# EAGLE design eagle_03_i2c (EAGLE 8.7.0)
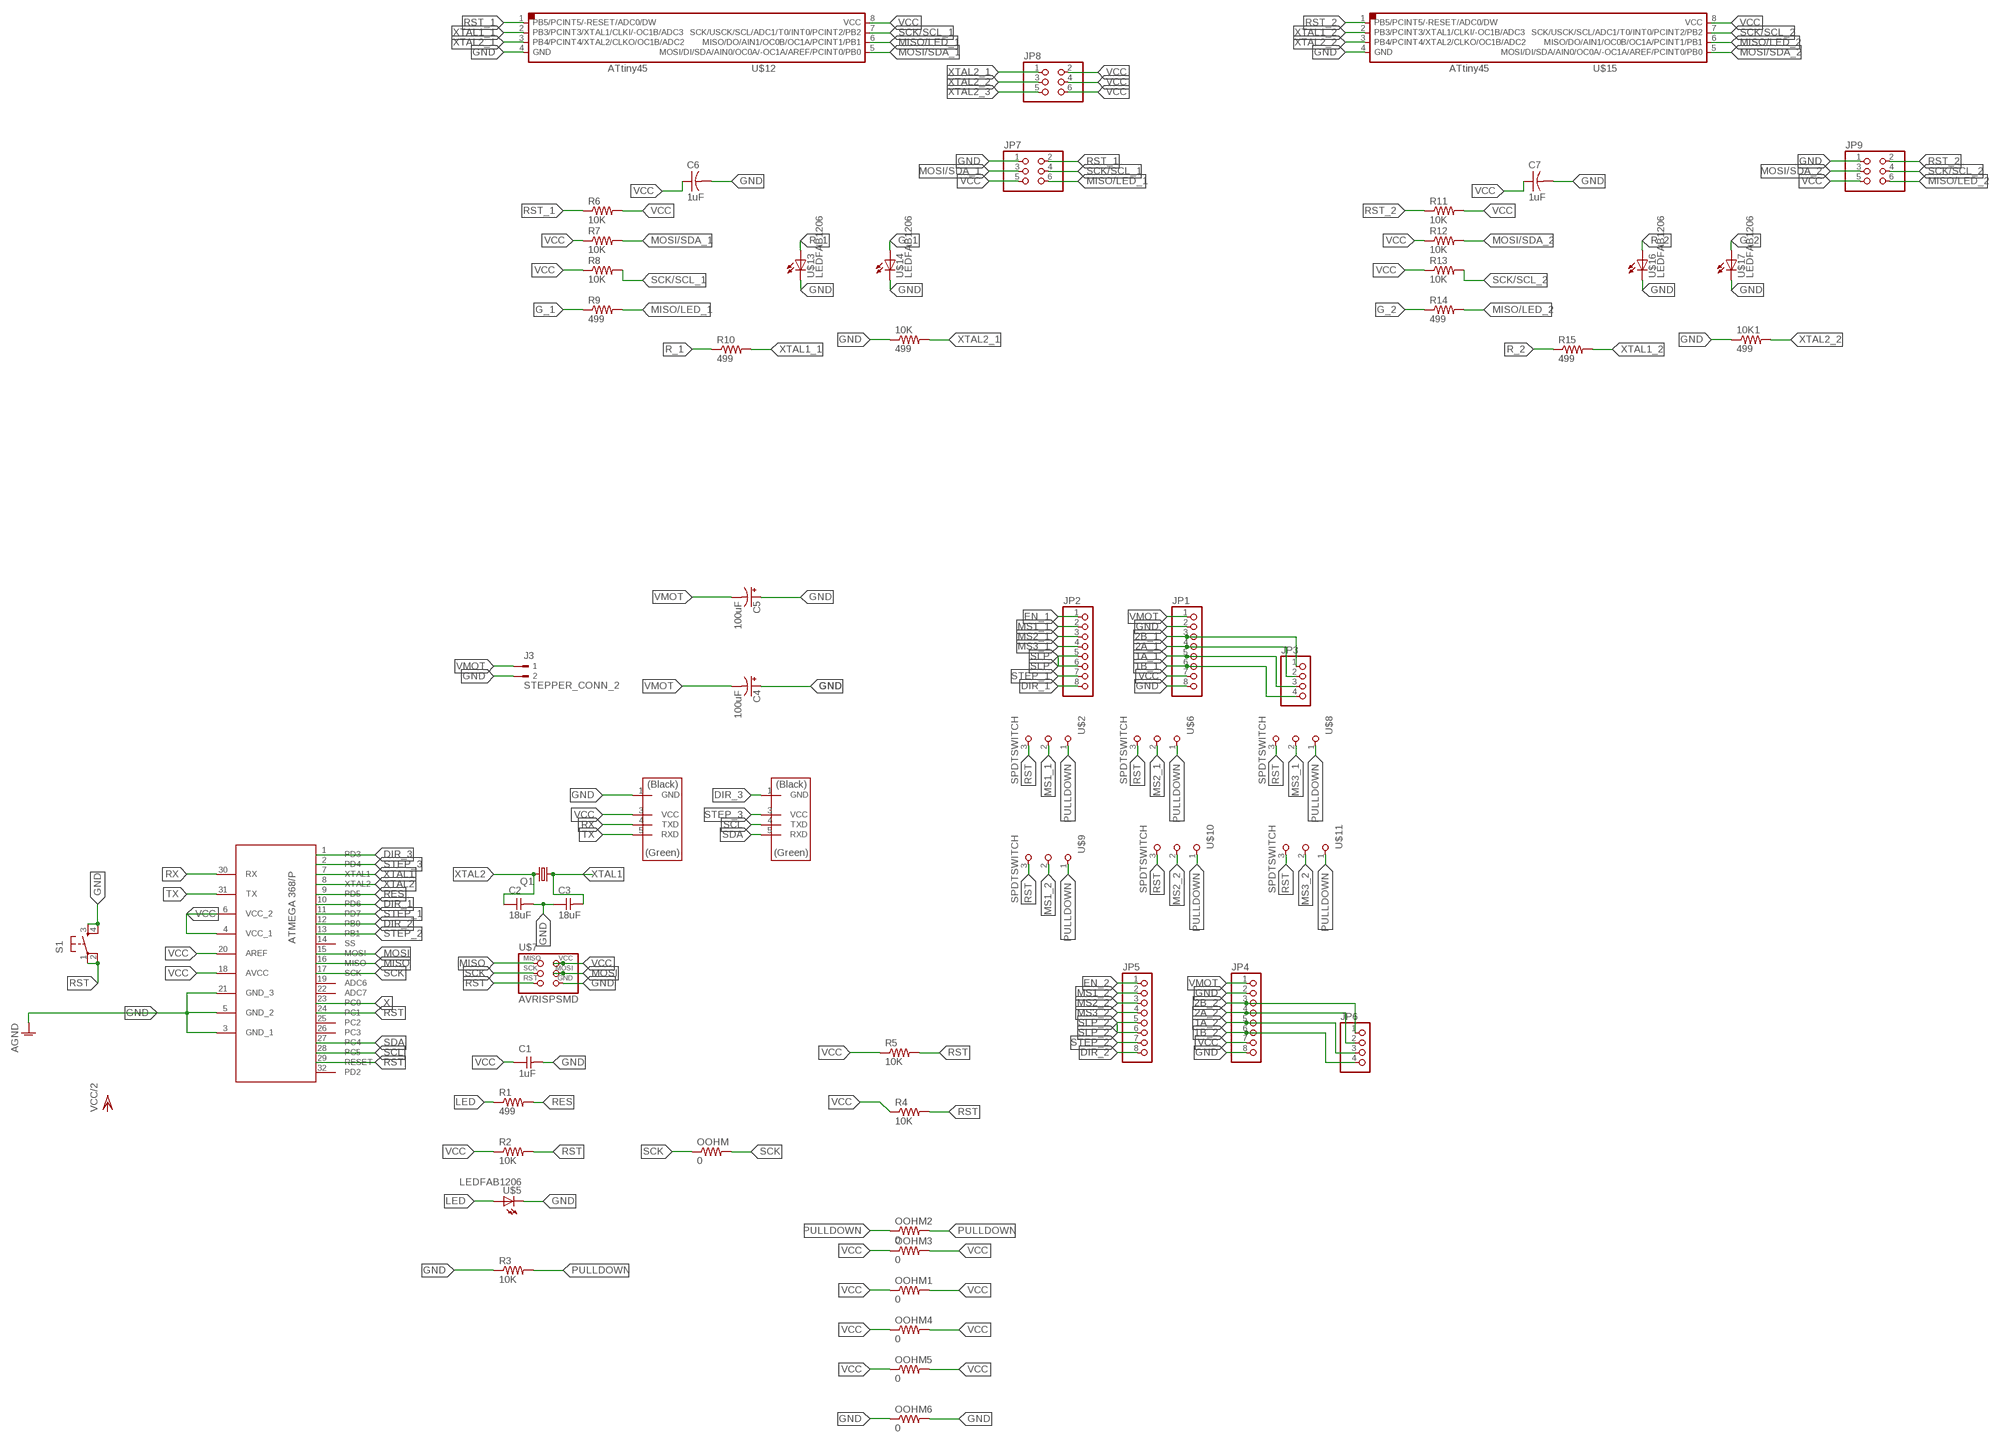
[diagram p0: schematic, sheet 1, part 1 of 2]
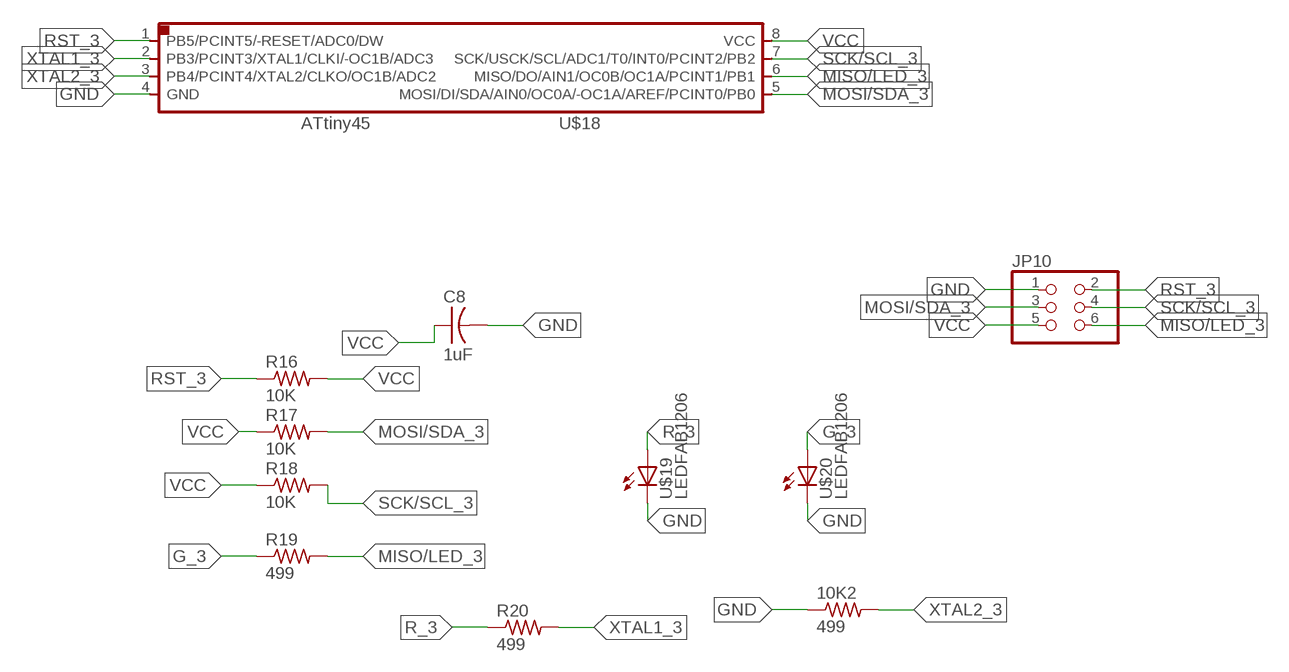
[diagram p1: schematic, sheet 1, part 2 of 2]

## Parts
10K  499  RES-US1206FAB  [R1206FAB]
10K1  499  RES-US1206FAB  [R1206FAB]
10K2  499  RES-US1206FAB  [R1206FAB]
C1  1uF  CAP-UNPOLARIZEDFAB  [C1206FAB]
C2  18uF  CAP-UNPOLARIZEDFAB  [C1206FAB]
C3  18uF  CAP-UNPOLARIZEDFAB  [C1206FAB]
C4  100uF  CAP_POLC  [PANASONIC_C]
C5  100uF  CAP_POLC  [PANASONIC_C]
C6  1uF  CAP-US1206FAB  [C1206FAB]
C7  1uF  CAP-US1206FAB  [C1206FAB]
C8  1uF  CAP-US1206FAB  [C1206FAB]
J3  STEPPER_CONN_2  PM5.08/2/90BLK  [WEIDMULLER_PM5.08_2]
JP1  PINHD-1X8  [1X08]
JP2  PINHD-1X8  [1X08]
JP3  PINHD-1X4  [1X04]
JP4  PINHD-1X8  [1X08]
JP5  PINHD-1X8  [1X08]
JP6  PINHD-1X4  [1X04]
JP7  PINHD-2X3-SMD  [2X03SMD]
JP8  PINHD-2X3-SMD  [2X03SMD]
JP9  PINHD-2X3-SMD  [2X03SMD]
JP10  PINHD-2X3-SMD  [2X03SMD]
OOHM  0  RES-US1206FAB  [R1206FAB]
OOHM1  0  RES-US1206FAB  [R1206FAB]
OOHM2  0  RES-US1206FAB  [R1206FAB]
OOHM3  0  RES-US1206FAB  [R1206FAB]
OOHM4  0  RES-US1206FAB  [R1206FAB]
OOHM5  0  RES-US1206FAB  [R1206FAB]
OOHM6  0  RES-US1206FAB  [R1206FAB]
Q1  CRYSTALSM49  [SM49]
R1  499  RES-US1206FAB  [R1206FAB]
R2  10K  RES-US1206FAB  [R1206FAB]
R3  10K  RES-US1206FAB  [R1206FAB]
R4  10K  RES-US1206FAB  [R1206FAB]
R5  10K  RES-US1206FAB  [R1206FAB]
R6  10K  RES-US1206FAB  [R1206FAB]
R7  10K  RES-US1206FAB  [R1206FAB]
R8  10K  RES-US1206FAB  [R1206FAB]
R9  499  RES-US1206FAB  [R1206FAB]
R10  499  RES-US1206FAB  [R1206FAB]
R11  10K  RES-US1206FAB  [R1206FAB]
R12  10K  RES-US1206FAB  [R1206FAB]
R13  10K  RES-US1206FAB  [R1206FAB]
R14  499  RES-US1206FAB  [R1206FAB]
R15  499  RES-US1206FAB  [R1206FAB]
R16  10K  RES-US1206FAB  [R1206FAB]
R17  10K  RES-US1206FAB  [R1206FAB]
R18  10K  RES-US1206FAB  [R1206FAB]
R19  499  RES-US1206FAB  [R1206FAB]
R20  499  RES-US1206FAB  [R1206FAB]
S1  6MM_SWITCH6MM_SWITCH  [6MM_SWITCH]
U$1  ATMEGA368  [ATMEGA328/P]
U$2  SPDTSWITCH  [SPDTSWITCH]
U$3  FTDI_2  [1X06SMD_2]
U$4  FTDI_2  [1X06SMD_2]
U$5  LEDFAB1206  [LED1206FAB]
U$6  SPDTSWITCH  [SPDTSWITCH]
U$7  AVRISPSMD  [2X03SMD]
U$8  SPDTSWITCH  [SPDTSWITCH]
U$9  SPDTSWITCH  [SPDTSWITCH]
U$10  SPDTSWITCH  [SPDTSWITCH]
U$11  SPDTSWITCH  [SPDTSWITCH]
U$12  ATTINY45SI  [SOIC8]
U$13  LEDFAB1206  [LED1206FAB]
U$14  LEDFAB1206  [LED1206FAB]
U$15  ATTINY45SI  [SOIC8]
U$16  LEDFAB1206  [LED1206FAB]
U$17  LEDFAB1206  [LED1206FAB]
U$18  ATTINY45SI  [SOIC8]
U$19  LEDFAB1206  [LED1206FAB]
U$20  LEDFAB1206  [LED1206FAB]

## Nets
1A_1: JP1.5 JP3.3
1A_2: JP4.5 JP6.3
1B_1: JP1.6 JP3.4
1B_2: JP4.6 JP6.4
2A_1: JP1.4 JP3.2
2A_2: JP4.4 JP6.2
2B_1: JP1.3 JP3.1
2B_2: JP4.3 JP6.1
DIR_1: JP2.8 U$1.10(PD6)
DIR_2: JP5.8 U$1.12(PB0)
DIR_3: U$1.1(PD3) U$3.1(GND)
EN_1: JP2.1
EN_2: JP5.1
G_1: R9.1 U$14.1(A)
G_2: R14.1 U$17.1(A)
G_3: R19.1 U$20.1(A)
GND: 10K1.1 10K2.1 10K.1 C1.2 C2.2 C3.1 C4.+ C5.+ C6.2 C7.2 C8.2 J3.2 JP1.2 JP1.8 JP4.2 JP4.8 JP7.1 JP9.1 JP10.1 OOHM6.1 OOHM6.2 R3.1 S1.3(S) S1.4(S1) U$1.3(GND_1) U$1.5(GND_2) U$1.21(GND_3) U$4.1(GND) U$5.2(C) U$7.6(GND) U$12.4(GND) U$13.2(C) U$14.2(C) U$15.4(GND) U$16.2(C) U$17.2(C) U$18.4(GND) U$19.2(C) U$20.2(C) ; supply symbol labelled AGND
LED: R1.1 U$5.1(A)
MISO: U$1.16(MISO) U$7.1(MISO)
MISO/LED_1: JP7.6 R9.2 U$12.6(MISO/DO/AIN1/OC0B/OC1A/PCINT1/PB1)
MISO/LED_2: JP9.6 R14.2 U$15.6(MISO/DO/AIN1/OC0B/OC1A/PCINT1/PB1)
MISO/LED_3: JP10.6 R19.2 U$18.6(MISO/DO/AIN1/OC0B/OC1A/PCINT1/PB1)
MOSI: U$1.15(MOSI) U$7.4(MOSI)
MOSI/SDA_1: JP7.3 R7.2 U$12.5(MOSI/DI/SDA/AIN0/OC0A/-OC1A/AREF/PCINT0/PB0)
MOSI/SDA_2: JP9.3 R12.2 U$15.5(MOSI/DI/SDA/AIN0/OC0A/-OC1A/AREF/PCINT0/PB0)
MOSI/SDA_3: JP10.3 R17.2 U$18.5(MOSI/DI/SDA/AIN0/OC0A/-OC1A/AREF/PCINT0/PB0)
MS1_1: JP2.2 U$2.2
MS1_2: JP5.2 U$9.2
MS2_1: JP2.3 U$6.2
MS2_2: JP5.3 U$10.2
MS3_1: JP2.4 U$8.2
MS3_2: JP5.4 U$11.2
PULLDOWN: OOHM2.1 OOHM2.2 R3.2 U$2.1 U$6.1 U$8.1 U$9.1 U$10.1 U$11.1
R_1: R10.1 U$13.1(A)
R_2: R15.1 U$16.1(A)
R_3: R20.1 U$19.1(A)
RES: R1.2 U$1.9(PD5)
RST: R2.2 R4.2 R5.2 S1.1(P) S1.2(P1) U$1.24(PC1) U$1.29(RESET) U$2.3 U$6.3 U$7.5(RST) U$8.3 U$9.3 U$10.3 U$11.3
RST_1: JP7.2 R6.1 U$12.1(PB5/PCINT5/-RESET/ADC0/DW)
RST_2: JP9.2 R11.1 U$15.1(PB5/PCINT5/-RESET/ADC0/DW)
RST_3: JP10.2 R16.1 U$18.1(PB5/PCINT5/-RESET/ADC0/DW)
RX: U$1.30(RX) U$4.4(TXD)
SCK: OOHM.1 OOHM.2 U$1.17(SCK) U$7.3(SCK)
SCK/SCL_1: JP7.4 R8.2 U$12.7(SCK/USCK/SCL/ADC1/T0/INT0/PCINT2/PB2)
SCK/SCL_2: JP9.4 R13.2 U$15.7(SCK/USCK/SCL/ADC1/T0/INT0/PCINT2/PB2)
SCK/SCL_3: JP10.4 R18.2 U$18.7(SCK/USCK/SCL/ADC1/T0/INT0/PCINT2/PB2)
SCL: U$1.28(PC5) U$3.4(TXD)
SDA: U$1.27(PC4) U$3.5(RXD)
SLP: JP2.5 JP2.6
SLP_2: JP5.5 JP5.6
STEP_1: JP2.7 U$1.11(PD7)
STEP_2: JP5.7 U$1.13(PB1)
STEP_3: U$1.2(PD4) U$3.3(VCC)
TX: U$1.31(TX) U$4.5(RXD)
VCC: C1.1 C6.1 C7.1 C8.1 JP1.7 JP4.7 JP7.5 JP8.2 JP8.4 JP8.6 JP9.5 JP10.5 OOHM1.1 OOHM1.2 OOHM3.1 OOHM3.2 OOHM4.1 OOHM4.2 OOHM5.1 OOHM5.2 R2.1 R4.1 R5.1 R6.2 R7.1 R8.1 R11.2 R12.1 R13.1 R16.2 R17.1 R18.1 U$1.4(VCC_1) U$1.6(VCC_2) U$1.18(AVCC) U$1.20(AREF) U$4.3(VCC) U$7.2(VCC) U$12.8(VCC) U$15.8(VCC) U$18.8(VCC)
VMOT: C4.- C5.- J3.1 JP1.1 JP4.1
X: U$1.23(PC0)
XTAL1: C3.2 Q1.1 U$1.7(XTAL1)
XTAL1_1: R10.2 U$12.2(PB3/PCINT3/XTAL1/CLKI/-OC1B/ADC3)
XTAL1_2: R15.2 U$15.2(PB3/PCINT3/XTAL1/CLKI/-OC1B/ADC3)
XTAL1_3: R20.2 U$18.2(PB3/PCINT3/XTAL1/CLKI/-OC1B/ADC3)
XTAL2: C2.1 Q1.2 U$1.8(XTAL2)
XTAL2_1: 10K.2 JP8.1 U$12.3(PB4/PCINT4/XTAL2/CLKO/OC1B/ADC2)
XTAL2_2: 10K1.2 JP8.3 U$15.3(PB4/PCINT4/XTAL2/CLKO/OC1B/ADC2)
XTAL2_3: 10K2.2 JP8.5 U$18.3(PB4/PCINT4/XTAL2/CLKO/OC1B/ADC2)
Unconnected: U$1.14(SS) U$1.19(ADC6) U$1.22(ADC7) U$1.25(PC2) U$1.26(PC3) U$1.32(PD2)

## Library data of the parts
10K 10K1 10K2 R6-R20 = 01fab:RES-US: Resistor (US Symbol)
C1-C3 = fab:CAP-UNPOLARIZED
C4 C5 = SparkFun-Capacitors:CAP_POL: Capacitor Polarized
C6-C8 = 01fab:CAP-US
J3 = WEIDMULLER-PM5.08_2_90BLK:PM5.08/2/90BLK: TERMINAL BLOCK, SIDE ENTRY, 2WAY; MPN: PM5.08/2/90 BLK; OC_FARNELL: 1131855; OC_NEWARK: 26M1980; PACKAGE: TH-R/A; SUPPLIER: WEIDMULLER
JP1 JP2 JP4 JP5 = pinhead:PINHD-1X8: PIN HEADER
JP3 JP6 = pinhead:PINHD-1X4: PIN HEADER
JP7-JP10 = 01fab:PINHD-2X3-SMD: PIN HEADER
OOHM OOHM1-OOHM6 R1-R5 = fab:RES-US: Resistor (US Symbol)
Q1 = crystal:CRYSTAL: CRYSTAL; OC_FARNELL: unknown; OC_NEWARK: unknown
S1 = fab:6MM_SWITCH: OMRON SWITCH
U$1 = Paul:ATMEGA368
U$2 U$6 U$8-U$11 = 01fab:SPDTSWITCH
U$3 = 01fab:FTDI_2
U$4 = fab:FTDI_2
U$5 = fab:LED: LED
U$7 = 01fab:AVRISP
U$12 U$15 U$18 = 01fab:ATTINY45
U$13 U$14 U$16 U$17 U$19 U$20 = 01fab:LED: LED

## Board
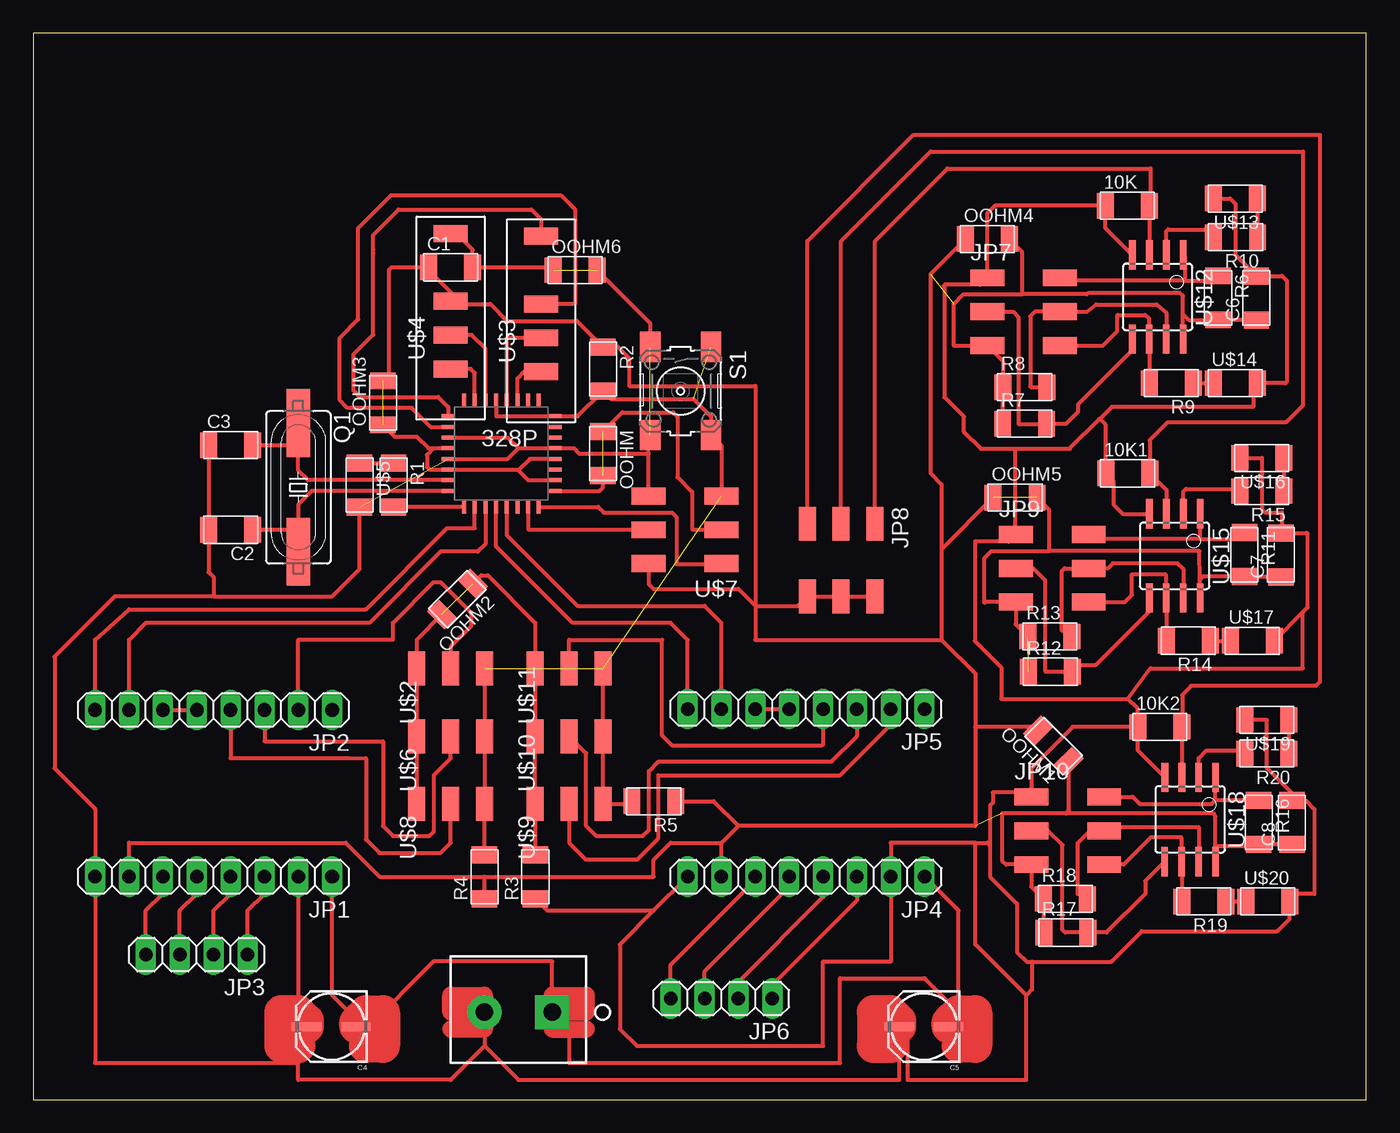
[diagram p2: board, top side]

Size 100 x 80 mm. Coordinates in mm from the lower left corner, seen from the top.
Outline: 0,0 100,0 100,80 0,80 0,0
Copper layers (1*16): Top 0.035mm / dielectric 1.5mm / Bottom 0.035mm
Design rules "default *": minimum track width 6mil, minimum drill 0.35mm, track to track 16mil, track to pad 16mil, pad to pad 16mil, via to via 16mil, smd to smd 16mil, copper to edge 40mil, drill to drill 6mil, minimum pad ring 10mil, minimum via ring 8mil, stop-mask expansion 4mil, vias tented up to drill 0mil, thermal gap 10mil

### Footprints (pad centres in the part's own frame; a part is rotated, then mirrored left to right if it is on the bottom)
R1206FAB = smd 1.27 x 1.905: 1 -1.651,0; 2 1.651,0
C1206FAB = smd 1.27 x 1.905: 1 -1.651,0; 2 1.651,0
PANASONIC_C = smd 2.2 x 0.65: + 1.9,-0.2; - -1.8,-0.2
WEIDMULLER_PM5.08_2 = drill 1.3 pad 2.54 square: 1 -2.54,0 | drill 1.3 pad 2.54: 2 2.54,0
1X08 = drill 1.016 long: 1 -8.89,0; 2 -6.35,0; 3 -3.81,0; 4 -1.27,0; 5 1.27,0; 6 3.81,0; 7 6.35,0; 8 8.89,0
1X04 = drill 1.016 long: 1 -3.81,0; 2 -1.27,0; 3 1.27,0; 4 3.81,0
2X03SMD = smd 2.54 x 1.27: 1 -2.54,2.54; 2 2.92,2.54; 3 -2.54,0; 4 2.92,0; 5 -2.54,-2.54; 6 2.92,-2.54
SM49 = smd 5.08 x 1.778: 1 -4.826,0; 2 4.826,0
6MM_SWITCH = smd 2.286 x 1.524: 1 -3.302,2.286; 2 3.302,2.286; 3 -3.302,-2.286; 4 3.302,-2.286
ATMEGA328/P = smd 1 x 0.3: 1 -4,2.8; 2 -4,2; 3 -4,1.2; 4 -4,0.4; 5 -4,-0.4; 6 -4,-1.2; 7 -4,-2; 8 -4,-2.8; 17 4,-2.8; 18 4,-2; 19 4,-1.2; 20 4,-0.4; 21 4,0.4; 22 4,1.2; 23 4,2; 24 4,2.8 | smd 0.3 x 1: 9 -2.8,-4; 10 -2,-4; 11 -1.2,-4; 12 -0.4,-4; 13 0.4,-4; 14 1.2,-4; 15 2,-4; 16 2.8,-4; 25 2.8,4; 26 2,4; 27 1.2,4; 28 0.4,4; 29 -0.4,4; 30 -1.2,4; 31 -2,4; 32 -2.8,4
SPDTSWITCH = smd 2.54 x 1.27: 1 0.38,2.54; 2 0.38,0; 3 0.38,-2.54
1X06SMD_2 = smd 2.54 x 1.27: 1 0,6.35; 3 0,1.27; 4 0,-1.27; 5 0,-3.81
LED1206FAB = smd 1.27 x 1.905: 1 -1.651,0; 2 1.651,0
SOIC8 = smd 0.5 x 2.2: 1 -1.905,-3.154; 2 -0.645,-3.154; 3 0.625,-3.154; 4 1.895,-3.154; 5 1.905,3.154; 6 0.635,3.154; 7 -0.635,3.154; 8 -1.905,3.154

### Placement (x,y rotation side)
10K  82.09,67.06 0 top
10K1  82.1,46.98 0 top
10K2  84.52,27.96 0 top
C1  31.31,62.44 0 top
C2  14.8,42.75 180 top
C3  14.8,49.1 0 top
C4  22.42,5.29 180 top
C5  66.87,5.29 180 top
C6  91.75,60.15 90 top
C7  93.61,40.87 90 top
C8  94.43,20.78 90 top
J3  36.39,6.56 180 top
JP1  13.53,16.72 180 top
JP2  13.53,29.23 180 top
JP3  12.26,10.87 180 top
JP4  57.98,16.72 180 top
JP5  57.98,29.3 180 top
JP6  51.63,7.57 180 top
JP7  74.11,59.11 0 top
JP8  60.61,40.66 270 top
JP9  76.26,39.86 0 top
JP10  77.42,20.17 0 top
OOHM  42.74,48.47 270 top
OOHM1  76.54,26.52 135 top
OOHM2  31.82,37.54 225 top
OOHM3  26.23,52.28 90 top
OOHM4  71.58,64.56 0 top
OOHM5  73.66,45.16 0 top
OOHM6  40.64,62.23 0 top
Q1  19.88,45.93 270 top
R1  27.03,46.1 270 top
R2  42.74,54.82 270 top
R3  37.66,16.72 90 top
R4  33.85,16.72 90 top
R5  46.55,22.38 180 top
R6  88.89,60.15 270 top
R7  74.38,50.71 0 top
R8  74.38,53.45 0 top
R9  85.37,53.76 180 top
R10  90.2,64.7 180 top
R11  90.87,40.88 270 top
R12  76.32,32.1 0 top
R13  76.28,34.74 0 top
R14  86.65,34.43 180 top
R15  92.16,45.66 180 top
R16  91.94,20.8 270 top
R17  77.46,12.53 0 top
R18  77.44,15.05 0 top
R19  87.82,14.86 180 top
R20  92.55,25.95 180 top
S1  48.56,53.16 270 top
U$1  35.12,48.47 0 top
U$2  31.31,31.96 90 top
U$3  38.1,58.42 0 top
U$4  31.31,58.63 0 top
U$5  24.47,46.1 270 top
U$6  31.31,26.88 90 top
U$7  49.09,42.75 180 top
U$8  31.31,21.8 90 top
U$9  40.2,21.8 90 top
U$10  40.2,26.88 90 top
U$11  40.2,31.96 90 top
U$12  84.36,60.21 180 top
U$13  90.19,67.6 180 top
U$14  90.17,53.75 0 top
U$15  85.63,40.79 180 top
U$16  92.17,48.14 180 top
U$17  91.45,34.42 0 top
U$18  86.79,21.01 180 top
U$19  92.54,28.48 180 top
U$20  92.61,14.86 0 top

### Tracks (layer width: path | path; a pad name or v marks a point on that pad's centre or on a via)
1A_1
  Top 0.305: 10.99,11.59 10.99,14.18 12.26,15.45 JP1.5
  Top 1.27: 12.19,17.46 12.26,17.39 JP1.5 | JP3.3 10.99,11.59
1A_2
  Top 0.305: 50.36,8.03 50.36,9.6 56.71,15.95
  Top 1.27: JP6.3 50.36,8.03 | JP4.5 56.71,15.95
1B_1
  Top 0.305: 8.45,11.59 8.45,14.18 9.72,15.45 9.72,16.27
  Top 1.27: JP1.6 9.72,16.27 | JP3.4 8.45,11.59
1B_2
  Top 0.305: 47.82,8.38 47.82,10.11 54.07,16.37
  Top 1.27: 47.88,6.77 47.82,6.84 JP6.4 47.82,8.38 | JP4.6 54.07,16.62 54.07,16.37
2A_1
  Top 0.305: 13.53,11.73 13.53,14.18 14.8,15.45 JP1.4
  Top 1.27: JP1.4 14.77,16.74 14.77,17.39 | JP3.2 13.53,11.73
2A_2
  Top 0.305: 59.25,16.06 59.25,15.19 52.9,8.84 52.9,7.89
  Top 1.27: JP6.2 52.9,7.89 | JP4.4 59.25,16.06
2B_1
  Top 0.305: 16.07,11.38 16.07,14.18 17.34,15.45 JP1.3
  Top 1.27: JP1.3 17.34,17.58 17.36,17.6 | JP3.1 16.07,11.38
2B_2
  Top 0.305: 61.79,16.34 61.79,14.94 55.44,8.59 55.44,7.82
  Top 1.27: JP6.1 55.44,7.82 | JP4.3 61.79,16.34
DIR_1
  Top 0.305: U$1.10 33.12,42.88 31.05,42.88 24.96,36.78 7.18,36.78 4.64,34.5 4.64,29.54
  Top 1.27: JP2.8 4.64,29.54
DIR_2
  Top 0.305: 49.09,29.61 49.09,34.5 47.82,35.77 40.47,35.77 34.72,41.51 U$1.12
  Top 1.27: JP5.8 49.09,29.61
DIR_3
  Top 0.305: U$1.1 31.12,51.96 30.37,52.71 24.48,52.71 24,53.22 24,55.88 25.5,57.38 25.5,63.5 25.5,63.8 25.5,64.87 27.4,66.77 37.37,66.77 38.1,66.04 U$3.1
EN_1
  Top 1.27: JP2.1 22.42,28.74 22.46,28.7
EN_2
  Top 1.27: JP5.1 66.95,29.22 66.95,28.64
G_1
  Top 0.305: R9.1 U$14.1
G_2
  Top 0.305: R14.1 U$17.1
G_3
  Top 0.305: R19.1 U$20.1
GND  (3 unrouted)
  Top 0.152: 32.96,62.49 C1.2 | 13.12,43.01 C2.2 | 13.12,48.87 C3.1
  Top 0.305: U$1.3 35.59,49.67 36.4,48.86 | 36.4,48.86 U$1.21 40.56,48.87 40.96,48.47 46.17,48.47 | U$1.5 35.6,48.07 36.4,48.86 | C3.1 C2.2 13.15,39.58 13.53,39.2 13.53,37.75 | U$7.6 46.17,48.47 | 46.17,48.47 46.17,49.75 S1.4 | 33.85,4.02 31.31,1.48 19.88,1.48 19.88,2.75 | 19.88,2.75 19.88,5.29 20.08,5.49 C4.+ | 19.88,16.41 19.88,6.56 | J3.2 33.85,4.02 | 33.85,4.02 36.39,1.48 64.96,1.48 C5.+ 65.6,4.86 65.6,1.48 74.49,1.48 74.49,7.83 | 70.68,19.26 70.68,11.64 74.49,7.83 | 70.68,19.26 64.33,19.26 JP4.2 | 13.53,37.75 22.42,37.75 24.47,39.8 U$5.2 | 4.64,16.2 4.64,2.75 19.88,2.75 | 46.55,14.18 49.03,16.66 | 64.33,16.34 64.33,10.37 59.25,10.37 59.25,4.02 45.28,4.02 44.01,5.29 44.01,11.64 46.55,14.18 | R3.1 38.55,14.18 46.55,14.18 | 13.53,37.75 6.11,37.75 1.59,33.23 1.59,24.84 4.64,21.8 JP1.8 | U$4.1 31.75,64.98 32.96,63.77 C1.2 38.78,62.44 OOHM6.1 | U$13.2 89.8,67.6 90.2,67.21 90.2,63.4 91.75,61.84 C6.2 93.69,61.8 94.03,61.46 94.03,53.84 93.94,53.76 U$14.2 91.49,53.42 91.53,51.97 80.91,51.97 80.01,51.07 | 73.66,48.84 71.08,48.84 69.83,50.1 69.83,51.23 68.35,52.7 68.35,60.97 68.28,61.04 68.37,61.13 71.05,61.13 JP7.1 71.57,66.49 72.14,67.06 10K.1 80.44,65.39 U$12.4 | 73.66,48.84 77.75,48.84 | 77.75,48.84 77.78,48.84 | 77.75,48.84 79.97,51.07 80.01,51.07 | U$16.2 92.17,48.14 92.18,48.15 92.18,44.28 92.42,44.05 93.69,44.05 93.69,42.6 C7.2 95.54,42.52 95.59,42.47 95.59,36.91 95.25,36.57 | U$15.4 81.76,43.94 81.05,44.65 81.05,46.39 10K1.1 80.45,50.62 80.01,51.07 | 95.25,36.57 U$17.2 | U$18.4 82.86,26.2 10K2.1 | JP10.1 74.88,23.39 | U$19.2 90.91,28.46 92.56,28.46 92.56,24.88 94.43,23.01 C8.2 95.46,22.43 96.12,21.77 96.12,15.42 94.83,15.42 U$20.2 94.26,13.56 93.32,12.62 83.16,12.62 80.88,10.34 74.93,10.34
  Top 0.305: JP10.1 74.54,23.04 71.99,23.04 71.99,22.27 71.78,22.05 71.78,19.05 | 71.78,19.05 71.78,16.72 73.81,14.69 73.81,11.06 74.53,10.34 74.93,10.34 | 10K2.1 77.99,27.96 74.87,24.83 74.87,22.72 JP10.1 | 73.66,48.84 73.66,42.46 JP9.1 73.18,41.86 70.66,41.86 70.65,41.87 | 82.13,30.06 72.62,30.06 72.62,32.42 70.61,34.43 70.65,34.46 70.65,41.87 | 95.25,36.57 95.25,32.36 83.82,32.36 82.13,30.06 | 10K2.1 82.86,29.33 82.13,30.06 | 74.93,10.34 74.93,8.27 74.49,7.83 | 70.68,19.26 71.57,19.26 71.78,19.05 | OOHM6.2 46.28,58.24 S1.3 | 70.64,41.87 70.65,41.87
  Top 0.406: JP1.8 4.26,16.34 4.09,16.34 4.16,16.41 4.16,17.04 5.06,17.04 5.13,16.97 5.13,16.7 4.64,16.2
  Top 1.27: J3.2 31.31,6.56 31.31,7.83 33.85,7.83 33.85,5.29 31.31,5.29 | JP1.2 19.88,16.41 | JP4.8 49.03,16.66 | JP4.2 64.33,16.34
  Top 2.54: C4.+ 20.52,5.92 19.88,6.56 18.61,6.56 18.61,4.02 19.88,4.02 | C5.+ 64.97,5.92 64.33,6.56 63.06,6.56 63.06,4.02 64.33,4.02
LED
  Top 0.305: U$5.1 R1.1
MISO
  Top 0.305: U$1.16 42.37,44.47 42.81,44.03 47.92,44.03 48.24,43.72 48.24,40.19 48.25,40.18 51.6,40.18 U$7.1
MISO/LED_1
  Top 0.305: JP7.6 80.25,56.57 81.33,57.65 81.35,58.87 83.42,58.87 83.72,58.6 U$12.6 R9.2
MISO/LED_2
  Top 0.305: JP9.6 81.88,37.32 82.43,37.87 82.43,39.41 84.9,39.41 84.97,39.34 84.97,37.66 U$15.6 R14.2
MISO/LED_3
  Top 0.305: JP10.6 81.81,17.63 83.84,19.66 86.12,19.66 86.16,19.62 U$18.6 86.16,14.86 R19.2
MOSI
  Top 0.305: U$1.15 37.12,42.83 37.18,42.77 46.15,42.77 U$7.4
MOSI/SDA_1
  Top 0.305: U$12.5 82.45,56.23 78.4,52.18 78.4,51.61 77.52,50.73 76.25,50.73 | 76.25,50.73 76.05,50.73 R7.2 | JP7.3 73.51,59.11 73.92,58.7 73.92,52.27 73.92,52.26 73.92,50.7 76.22,50.7 76.25,50.73
MOSI/SDA_2
  Top 0.305: JP9.3 75.02,39.86 75.91,38.97 75.91,32.16 75.98,32.09 75.99,32.1 R12.2 78.48,32.62 79.72,32.62 83.73,36.63 U$15.5
MOSI/SDA_3
  Top 0.305: JP10.3 76.13,20.17 77.21,19.09 77.21,12.72 77.4,12.53 R17.2 80.52,12.53 83.42,15.42 83.42,16.39 U$18.5
MS1_1
  Top 0.305: 19.88,29.68 19.88,34.5 26.99,34.5 26.99,35.77 30.04,38.81 30.55,38.81 32.83,36.53 32.83,35.51 31.31,33.99 U$2.2
  Top 1.27: JP2.2 19.88,29.68
MS1_2
  Top 0.305: U$9.2 40.2,19.26 41.47,17.99 45.28,17.99 46.91,19.61 46.91,24.34 60.52,24.34 64.33,28.15 64.33,29.05
  Top 1.27: JP5.2 64.33,29.05
MS2_1
  Top 0.305: 17.34,28.91 17.34,26.88 26.23,26.88 26.23,20.53 26.99,19.76 29.71,19.76 30.04,20.09 30.04,24.34 31.31,25.61 U$6.2
  Top 1.27: JP2.3 17.34,28.91
MS2_2
  Top 0.305: JP5.3 61.79,29.42 | U$10.2 41.47,25.99 41.47,20.53 42.23,19.76 45.72,19.76 46.19,20.24 46.19,24.63 46.91,25.35 59.9,25.35 61.79,27.25 61.79,28.98
  Top 1.27: JP5.3 61.79,28.98
MS3_1
  Top 0.305: 14.8,28.5 14.8,25.62 23.69,25.62 24.96,25.61 24.96,19.51 25.98,18.49 30.55,18.49 31.31,19.26 U$8.2
  Top 1.27: JP2.4 14.8,28.5
MS3_2
  Top 0.305: U$11.2 40.2,34.5 47.18,34.5 47.18,27.32 47.97,26.54 59.13,26.54 59.25,26.66 59.25,29.05
  Top 1.27: JP5.4 59.25,29.05
PULLDOWN  (1 unrouted)
  Top 0.305: U$8.1 U$6.1 U$2.1 28.77,34.5 OOHM2.2 | R3.2 U$9.1 U$10.1 U$11.1 37.66,35.77 34.1,39.32 33.59,39.32 OOHM2.1
R_1
  Top 0.305: U$13.1 91.84,64.71 R10.1
R_2
  Top 0.305: U$16.1 93.82,45.67 R15.1
R_3
  Top 0.305: U$19.1 R20.1
RES
  Top 0.305: U$1.9 28.32,44.47 R1.2
RST  (3 unrouted)
  Top 0.305: U$7.5 51.63,49.08 S1.2 50.85,51.25 49.53,52.57 43.33,52.57 R2.2 40.84,51.27 U$1.24 34.74,51.27 34.72,51.28 U$1.29 | U$2.3 U$6.3 U$8.3 R4.2 | U$11.3 U$10.3 U$9.3 44.69,22.18 R5.2
RST_1
  Top 0.305: U$12.1 86.41,63.22 86.41,61.46 | 86.41,61.46 77.22,61.46 JP7.2 | 86.41,61.46 88.55,61.46 R6.1
RST_2
  Top 0.305: U$15.1 87.54,42.05 | 87.54,42.05 79.53,42.05 JP9.2 | 87.54,42.05 90.39,42.05 R11.1
RST_3
  Top 0.305: JP10.2 82.48,22.71 83.02,22.17 88.39,22.17 88.64,22.42 | 88.64,22.42 88.68,22.42 88.68,24.14 U$18.1 | R16.1 88.67,22.45 88.64,22.42
RX
  Top 0.305: U$4.4 32.89,57.36 33.92,56.33 U$1.30
SCK  (1 unrouted)
  Top 0.305: U$1.17 42.48,45.67 42.74,45.93 OOHM.2 | U$7.3 51.61,42.77 49.43,42.77 49.43,45.59 48.33,46.69 48.33,51.23 48,51.56 44.18,51.56 OOHM.1
SCK/SCL_1
  Top 0.305: U$12.7 85,59.06 84.29,59.65 79.74,59.65 79.03,59.11 JP7.4 75.14,59.11 74.79,58.76 74.79,53.52 74.86,53.45 R8.2
SCK/SCL_2
  Top 0.305: U$15.7 86.27,39.81 85.84,40.23 80.98,40.23 80.61,39.86 JP9.4 77.37,39.86 77.18,39.66 77.18,35.16 77.52,35.16 R13.2
SCK/SCL_3
  Top 0.305: U$18.7 87.44,20.44 80.61,20.44 JP10.4 79.27,20.17 78.34,19.23 78.34,15.42 78.72,15.42 R18.2
SCL
  Top 0.305: U$3.4 35.56,57.15 35.52,57.11 U$1.28
SDA
  Top 0.305: U$1.27 36.32,54.1 36.83,54.61 U$3.5
SLP
  Top 0.305: 9.88,29.23 12.12,29.23
  Top 1.27: JP2.5 12.12,29.23 | JP2.6 9.88,29.23
SLP_2
  Top 0.305: 54.31,29.3 56.61,29.3
  Top 1.27: JP5.5 56.61,29.3 | JP5.6 54.31,29.3
STEP_1
  Top 0.305: U$1.11 33.92,41.68 33.34,41.1 30.55,41.1 25.21,35.77 8.45,35.77 7.18,34.5 7.18,29.4
  Top 1.27: JP2.7 7.18,29.4
STEP_2
  Top 0.305: U$1.13 35.52,42.35 40.83,37.04 50.36,37.04 51.63,35.77 51.63,29.54
  Top 1.27: JP5.7 51.63,29.54
STEP_3
  Top 0.305: U$1.2 29.82,50.47 28.39,51.9 23.56,51.9 22.99,52.47 22.99,57.15 24.38,58.55 24.38,65.4 26.83,67.84 39.59,67.84 40.38,67.05 40.45,66.99 40.64,66.79 40.64,59.69 U$3.3
TX
  Top 0.305: U$4.5 32.81,54.82 33.12,54.51 U$1.31
VCC  (5 unrouted)
  Top 0.305: 29.66,61.55 29.66,62.23 | 29.66,62.23 C1.1 26.88,62.44 26.67,62.23 26.67,54.37 OOHM3.2 | U$1.20 37.26,48.07 36.46,47.27 | 36.46,47.27 36.39,47.2 37.12,46.47 U$1.18 | 36.46,47.27 U$1.6 29.71,47.27 29.53,47.45 29.53,48.36 30.04,48.87 | 30.04,48.87 29.64,48.87 28.77,49.74 27.12,49.74 OOHM3.1 | 30.04,48.87 U$1.4 | 70.68,27.94 70.68,31.96 68.14,34.5 | 70.68,27.94 70.68,20.53 52.9,20.53 | 51.63,17.18 51.63,19.26 | 51.63,19.26 52.9,20.53 | 7.18,17.25 7.18,19.26 23.43,19.26 25.98,16.72 33.85,16.72 | U$7.2 46.17,38.69 46.55,38.31 52.9,38.31 54.17,37.04 | 54.17,37.04 54.17,34.5 68.14,34.5 | R4.1 33.85,16.72 | 54.17,37.04 54.17,53.55 44.71,53.55 44.71,55.62 43.86,56.47 R2.1 40.79,58.42 35.56,58.42 34.29,59.69 31.52,59.69 U$4.3 31.31,60.58 29.66,62.23 | 51.63,19.26 47.82,19.26 46.55,17.99 46.55,16.72 33.85,16.72 | R5.1 51.05,22.38 52.9,20.53 | U$12.8 86.26,58.92 | 86.26,58.92 86.26,60.31 85.98,60.51 79.19,60.51 79.02,60.42 74.18,60.42 | R7.1 R8.1 72.73,55.42 JP7.5 71.56,56.56 69.08,56.56 69.06,56.58 69.06,59.69 69.79,60.42 74.18,60.42 | C6.1 R6.2 86.68,58.5 86.26,58.92 | U$15.8 87.51,37.66 87.5,38.97 | 87.5,38.97 87.49,41.15 76.2,41.15 | 87.5,38.97 87.76,39.23 R11.2 93.6,39.23 C7.1 | R13.1 73.72,35.66 JP9.5 71.41,37.32 71.36,37.27 71.36,40.64 71.86,41.15 76.2,41.15 | R17.1 75.79,12.55 R18.1 74.88,15.96 JP10.5 72.97,17.63 72.68,17.92 72.68,21.45 72.67,21.46 77.47,21.46 | C8.1 94.41,19.15 92.71,19.15 | 92.71,19.15 R16.2 | U$18.8 88.7,19.05 | 88.7,19.05 88.7,21.24 88.57,21.46 77.47,21.46 | 77.47,21.46 77.7,21.69 OOHM1.1 | OOHM1.2 75.11,27.94 70.68,27.94 | OOHM5.2 76.2,44.27 76.2,41.15 | OOHM5.1 68.14,41.29
  Top 0.305: 68.14,41.29 68.14,34.5 | OOHM4.2 74.18,63.62 74.18,60.42 | OOHM4.1 67.31,61.94 67.31,46.99 68.14,46.16 68.14,41.29 | 88.7,19.05 92.61,19.05 92.71,19.15 | 54.17,37.04 57.37,37.04 JP8.6 JP8.4 JP8.2
  Top 1.27: JP1.7 7.18,17.25 | JP4.7 51.63,17.18
VMOT
  Top 0.305: 24.76,5.49 22.42,7.83 JP1.1 | 69.41,6.56 66.87,9.1 60.52,9.1 60.52,2.75 40.2,2.75 40.2,5.29 J3.1 38.93,10.37 30.04,10.37 24.96,5.29 24.76,5.49 | 69.41,6.56 69.41,5.29 68.87,5.29 C5.- | 69.41,6.56 69.41,14.18 66.89,16.7 | C4.- 24.76,5.49
  Top 1.27: 38.93,7.83 41.47,7.83 41.47,6.56 J3.1 38.93,5.29 41.47,5.29 | JP1.1 22.53,16.82 22.53,17.32 | JP4.1 66.89,16.7
  Top 2.54: C4.- 24.22,5.82 24.96,6.56 26.23,6.56 26.23,4.02 24.96,4.02 | C5.- 68.67,5.82 69.41,6.56 70.68,6.56 70.68,4.02 69.41,4.02
XTAL1
  Top 0.305: U$1.7 20.61,46.47 19.88,47.2 19.88,49.74 | 19.88,49.74 Q1.1 | C3.2 19.24,49.1 19.88,49.74
XTAL1_1
  Top 0.305: U$12.2 85,65.13 85.14,65.27 88.95,65.27 88.95,65.1 R10.2
XTAL1_2
  Top 0.305: U$15.2 86.28,45.62 86.48,45.82 90.35,45.82 R15.2
XTAL1_3
  Top 0.305: U$18.2 87.44,25.61 88.01,26.18 90.67,26.18 R20.2
XTAL2
  Top 0.305: U$1.8 20.89,45.67 19.88,44.66 19.88,42.12 | 19.88,42.12 Q1.2 | C2.1 19.24,42.75 19.88,42.12
XTAL2_1
  Top 0.305: U$12.3 83.74,63.37 10K.2 83.82,67.14 83.82,69.85 68.58,69.85 63.15,64.42 JP8.1
XTAL2_2
  Top 0.305: U$15.3 85.01,45.73 10K1.2 83.75,49.47 85.09,50.8 93.98,50.8 95.25,52.07 95.25,71.12 67.31,71.12 60.61,64.42 JP8.3
XTAL2_3
  Top 0.305: U$18.3 10K2.2 86.19,27.99 86.19,30.35 86.88,31.04 96.22,31.04 96.52,31.34 96.52,72.39 66.04,72.39 58.07,64.42 JP8.5 | U$18.3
